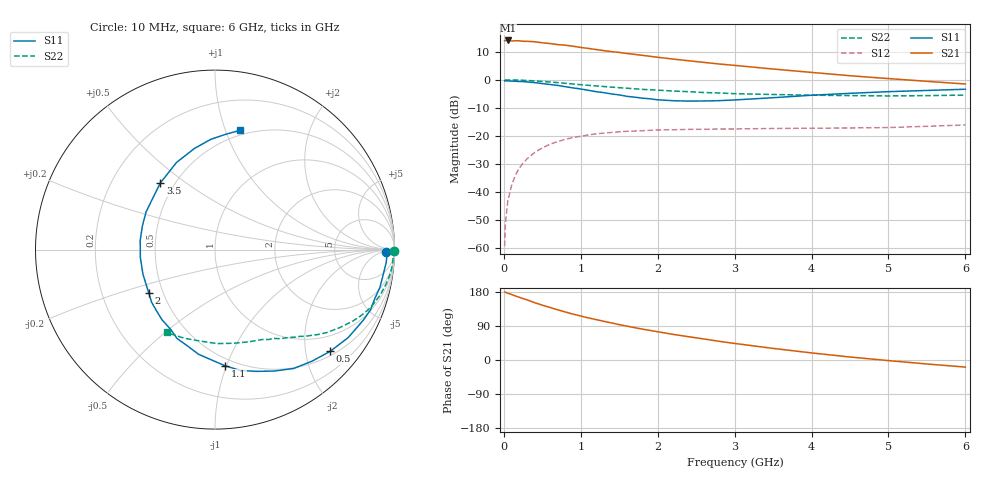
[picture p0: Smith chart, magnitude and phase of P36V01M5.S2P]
! SIEMENS Small Signal Semiconductors
! BFP181
! Si NPN RF Bipolar Junction Transistor in SOT143
! VCE = 6 V  IC = 1.5 mA
! Common Emitter S-Parameters:  March  1996
# GHz  S  MA  R  50
!  f  S11  S21  S12  S22
! GHz  MAG  ANG  MAG  ANG  MAG  ANG  MAG  ANG
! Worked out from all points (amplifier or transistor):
!   36 points, 10 MHz to 6 GHz, reference 50 ohm
!   highest |S21| = 14.0 dB at 50 MHz (marker M1)
!   |S21| within 3 dB of that: start of sweep to 1.141 GHz
!   unconditionally stable (mu >= 1): 2.81 GHz to end of sweep
!   at 250 MHz: K = 0.10, MSG = 21.7 dB, |S12| = -29.7 dB
!   at 1.4 GHz: K = 0.56, MSG = 14.4 dB, |S12| = -18.7 dB
!   at 6 GHz: K = 1.20, MAG = 4.6 dB, |S12| = -16.0 dB
!   S11 on the Smith chart (normalised r, x): 10 MHz: 37, -12; 500 MHz: 0.59, -2.52; 1.1 GHz: 0.44, -0.99; 2 GHz: 0.42, -0.25; 3.5 GHz: 0.42, +0.40; 6 GHz: 0.46, +1.13
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0.01  0.9527 -0.9  4.947 179.4  0.0011 85.6  0.9978 -0.3
0.02  0.9582 -1.8  4.988 179.0  0.0027 85.3  0.9903 -0.7
0.05  0.9568 -4.2  5.003 176.3  0.0068 91.2  0.9942 -2.0
0.1  0.9475 -8.4  4.902 172.9  0.0131 82.6  0.9931 -4.0
0.2  0.9314 -16.9  4.933 165.5  0.0268 78.9  0.9856 -7.8
0.4  0.8896 -33.4  4.75 151.3  0.051 69.0  0.9549 -15.3
0.5  0.8565 -41.4  4.546 144.7  0.0615 63.8  0.9352 -18.7
0.6  0.8241 -48.9  4.411 138.6  0.0715 59.3  0.914 -21.8
0.8  0.7528 -64.0  4.116 126.6  0.0873 51.4  0.866 -27.3
0.9  0.7163 -71.3  3.952 121.1  0.094 47.7  0.8406 -29.8
1.1  0.6494 -85.1  3.611 111.0  0.1046 41.4  0.7972 -34.2
1.3  0.5904 -98.9  3.299 102.1  0.1127 35.9  0.7592 -38.0
1.5  0.5381 -113.2  3.067 93.3  0.1186 31.6  0.7222 -41.3
1.8  0.4717 -133.7  2.721 81.5  0.1241 26.4  0.6761 -45.6
2  0.4404 -147.1  2.514 74.6  0.1279 23.1  0.6539 -48.3
2.2  0.4242 -161.1  2.336 67.6  0.129 20.5  0.6311 -51.2
2.8  0.4253 162.3  1.908 49.3  0.1334 14.6  0.5828 -59.3
3.5  0.48 129.5  1.553 30.6  0.1362 10.7  0.5476 -69.7
4  0.5307 113.8  1.353 18.7  0.1378 8.4  0.5321 -78.7
4.5  0.5746 101.6  1.181 7.9  0.139 6.9  0.5238 -88.6
5.5  0.646 84.5  0.939 -10.5  0.1489 7.3  0.5228 -109.4
6  0.6797 78.0  0.841 -18.7  0.1577 6.4  0.5343 -120.2
